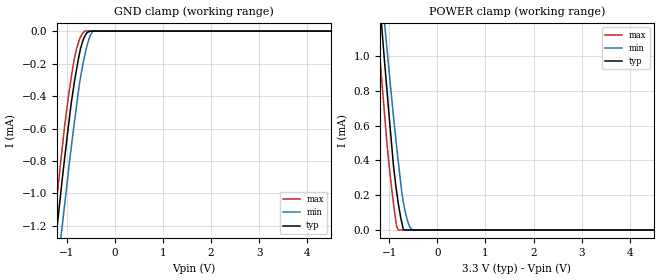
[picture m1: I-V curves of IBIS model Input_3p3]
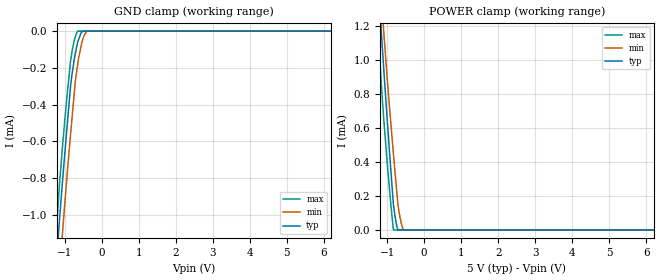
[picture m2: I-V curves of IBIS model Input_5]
|Texas Instruments Incorporated
|Low-Power, Low-Glitch, 12-Bit DAC
| Marketing part#   Digital Voltage Range   Package-type   #pins
| DAC7554IDGS   2.7 to 5.5V   MSOP   10
| DAC7554IDGSG4   2.7 to 5.5V   MSOP   10
| DAC7554IDGSR   2.7 to 5.5V   MSOP   10
| DAC7554IDGSRG4   2.7 to 5.5V   MSOP   10
[IBIS Ver]   3.2
[File name]   dac7554.ibs
|SIMDE Ver   V2.0 - 201002 - RHL4 - Build 372
[File Rev]   1.2
[Date]   07/20/2010
[Source]
|   Texas Instruments Incorporated.
|   Analog-eLab Design Center, HPA
|   12500 TI Blvd
|   Dallas, TX -75243
|   e-mail: elab_ibis@list.ti.com
|   -Model generated from simulations in TISPICE
[Notes]   Revision History:
|   Rev 1.0: 06/30/2010
|   - Initial version of the model
|   - Model generated from simulations in TISPICE
|   - Model matched to SPICE simulation
|   - Model names with a trailing 3p3 contains the model for
|   3.3V [3.0V and 3.6V]. Model names with trailing 5v contains
|   the model for 5.0V [4.5V and 5.5V] operation.
|   - C_comp although listed in numerical order of value are
|   obtained from varying PVT conditions. For PVT conditions for
|   each specific value refer the buffer description under
|   respective [Model]. IBIS model user is responsible for using
|   appropriate C_comp to simulate for Signal Integrity.
|   Rev 1.1: 07/08/2010
|   -Updated the ibis file with the changed package details.
|   -Removed the C_comp[ON state] and C-comp[OFF state] lines
|   from the Input_3p3 and Input_5 models in ibis file.
|   Rev 1.2: 07/20/2010
|   -Updated Vinl and Vinh parameters and added [model spec]
|   for the same as per datasheet
|   -Removed extra data points beyond -VDD(typ) and 2*VDD(typ)
|   in IV data
|   -added note on junction temperature
[Disclaimer]
| This model is designed as an aid for customers of Texas Instruments.
| TI and its licensors and suppliers make no warranties, either expressed
| or implied, with respect to this  model, including the warranties of
| merchantability or fitness for a particular purpose. The model is
| provided solely on an "as is" basis. The entire risk as to its quality
| and performance is with the customer.
[Copyright]
|(C) Copyright 2010 Texas Instruments Incorporated.All rights reserved.
|   DAC7554
[Component]   DAC7554
[Manufacturer]  TI
[Package]   | 10 MSOP - DGS package
|   typ   min   max
R_pkg   0.041315   0.02808   0.05455
L_pkg   1.39000nH   1.26021nH   1.51979nH
C_pkg   0.267465pF   0.23984pF   0.29509pF
|-------------------------PINS------------------------------------------------
[Pin]  signal_name model_name   R_pin   L_pin   C_pin
1   VOUTA   NC   0.02817   1.28097nH   0.25671pF
2   VOUTB   NC   0.02808   1.26021nH   0.29509pF
3   GND   GND   0.02799   1.24914nH   0.29579pF
4   VOUTC   NC   0.02815   1.26626nH   0.29308pF
5   VOUTD   NC   0.02817   1.28230nH   0.25594pF
6   SCLK   INPUT   0.05455   1.51979nH   0.23984pF
7   DIN   INPUT   0.05147   1.44516nH   0.27280pF
8   VDD   POWER   0.02787   1.25283nH   0.29098pF
9   _SYNC   INPUT   0.05142   1.44733nH   0.27042pF
10   REFIN   NC   0.02844   1.28864nH   0.25632pF
|   Model Selectors
[Model Selector]   INPUT
Input_3p3   3.3V digital input
Input_5   5.0V digital input
| Models and submodels in the file (2): Input_3p3 (Input), Input_5 (Input)
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|NOTES   Model INPUT split into two Models Input_3p3 and Input_5
|   to accomodate vast voltage range of 2.7V - 5.5V
|   INPUT_3p3 operates in voltage range of 3 - 3.3 - 3.6
|   INPUT_5 operates in voltage range of 4.5 - 5 - 5.5
|   The max pin frequency for Model INPUT is 50MHz.
|   INPUT 3.3V Model
[Model]   Input_3p3
Model_type   Input
Vinl = 0.99
Vinh = 2.31
|   typ   min   max
|   (nom PVT)   (Fast PVT)   (slow PVT)
C_comp   5.147e-13   4.725e-13   5.286e-13
| Where   nom PVT is Nominal Process, 3.3V, 25C
|   Fast PVT is Strong Process, 3.6V, -40C
|   Slow PVT is Weak Process, 3.0V, 105C
[Model Spec]
Vinl   0.99   0.9   1.08
Vinh   2.31   2.1   2.52
[Voltage Range]   3.3   3   3.6
|Junction temperature
[Temperature Range]   25   105   -40
[Power Clamp Reference]   3.3   3   3.6
[GND Clamp Reference]   0   0   0
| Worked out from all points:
|   GND clamp passes 1 mA (typ) near -1.13 V on its own axis
|   POWER clamp passes 1 mA (typ) near -1.11 V on its own axis
[GND Clamp]
|   Voltage   I(typ)   I(min)   I(max)
-3.3V     -7.395mA   -7.4mA     -7.717mA
-1.332V   -1.571mA   -1.836mA   -1.406mA
-1.234V   -1.292mA   -1.569mA   -1.108mA
-1.128V   -1.003mA   -1.284mA   -808.9uA
-1.086V   -887uA     -1.174mA   -692.7uA
-906mV    -440.1uA   -712.5uA   -280.8uA
-794.4mV  -231.6uA   -453uA     -105.8uA
-712.8mV  -105.7uA   -282uA     -35.6uA
-630mV    -34.32uA   -152.3uA   -33.57nA
-528mV    -2.612uA   -38.29uA   0A
-448.8mV  0A         0A         0A
6.6V      0A         0A         0A
[POWER Clamp]
|   Voltage   I(typ)   I(min)   I(max)
-3.3V     8.989mA    8.1mA      8.682mA
-1.241V   1.459mA    1.614mA    1.149mA
-1.176V   1.234mA    1.418mA    926.1uA
-1.112V   1.012mA    1.228mA    710.7uA
-1.076V   891.2uA    1.12mA     588.3uA
-956.4mV  505.3uA    774.1uA    251.6uA
-848.4mV  221.6uA    483.2uA    21.35uA
-816mV    157.7uA    400.4uA    0A
-712.8mV  7.897uA    166.8uA    0A
-660mV    0A         92.42uA    0A
-514.8mV  0A         0A         0A
6.6V      0A         0A         0A
|   INPUT 5.0V Model
[Model]   Input_5
Model_type   Input
Vinl = 1.5
Vinh = 3.5
|   typ   min   max
|   (nom PVT)   (Fast PVT)   (slow PVT)
C_comp   4.942e-13   4.462e-13   5.078e-13
| Where   nom PVT is  Nominal Process, 5.0V, 25C
|   Fast PVT is Strong Process, 5.5V, -40C
|   Slow PVT is Weak Process, 4.5V, 105C
[Model Spec]
Vinl   1.5   1.35   1.65
Vinh   3.5   3.15   3.85
[Voltage Range]   5   4.5   5.5
| Junction temperature
[Temperature Range]   25   105   -40
[Power Clamp Reference]   5   4.5   5.5
[GND Clamp Reference]   0   0   0
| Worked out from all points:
|   GND clamp passes 1 mA (typ) near -1.13 V on its own axis
|   POWER clamp passes 1 mA (typ) near -1.11 V on its own axis
[GND Clamp]
|   Voltage   I(typ)   I(min)   I(max)
-5V       -12.51mA   -12.28mA   -13.26mA
-1.22V    -1.255mA   -1.532mA   -1.074mA
-1.139V   -1.03mA    -1.315mA   -834.4uA
-1.051V   -804.5uA   -1.083mA   -613.6uA
-952mV    -563.7uA   -831.7uA   -388.8uA
-836.5mV  -296.5uA   -556.2uA   -158.4uA
-748.5mV  -165.8uA   -357.2uA   -59.14uA
-707mV    -117.9uA   -266.3uA   -29.32uA
-650mV    -62.68uA   -185.9uA   -397.9nA
-536mV    -4.583uA   -63.2uA    0A
-391mV    0A         0A         0A
10V       0A         0A         0A
[POWER Clamp]
|   Voltage   I(typ)   I(min)   I(max)
-5V       15.3mA     13.54mA    14.99mA
-1.31V    1.704mA    1.824mA    1.398mA
-1.171V   1.214mA    1.403mA    908.1uA
-1.139V   1.105mA    1.309mA    797.4uA
-1.089V   941.7uA    1.162mA    649.5uA
-941mV    477.1uA    737.8uA    251uA
-825mV    141.6uA    435.7uA    0A
-740mV    24.52uA    227.6uA    0A
-707mV    0A         147.9uA    0A
-617mV    0A         38.28uA    0A
-549.5mV  0A         0A         0A
10V       0A         0A         0A
